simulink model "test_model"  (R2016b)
settings: Solver=VariableStepAuto  StartTime=0.0  StopTime=runtime  RelTol=1e-3
InitFcn:
  | clear mex
  | delete test_model_sfun.mexw64
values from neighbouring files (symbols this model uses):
  delta_T = 4 * [ 0,  0,  2.351e-4 ]    [modelParameters.m]
  Delta_T = cell(1,4)    [modelParameters.m]
  F_D = 1*randn(3,1)    [modelParameters.m]
  g = 9.81    [modelParameters.m]    (also in analyzeIMU_data.m = 9.8; getMomentOfInertia.m = 9.80665)
  Gamma_H = cell(1,4)    [modelParameters.m]
  have_motor_transient = 1    [modelParameters.m]
  height_controlled_o = (((Rm*If        + (((omega0_o * 2 * Rm * Kv * Kq      * Kd + 1)^2) - 1)/(4* Rm*Kv^2*Kq      * Kd))/Vb)*(Pmax - Pmin) + Pmin)    [modelParameters.m]
  i_0 = cell(1,4)    [modelParameters.m]
  If = 0.3836    [modelParameters.m]    (also in thrustDragConstantCalculations.m = [If0; If1; If2; If3]; Kd_error.m = I_0 * sign(rotor_speed_0) + I_1 * rotor_speed_0 + I_2 * roto)
  J = diag([ 0.0130 0.0140 0.0285 ])    [modelParameters.m]    (also in J_calc_bifilar.m = (16*pi^2*L./(m*g.*D.^2))\(t./n).^2)
  J_L = m_L/12*diag([y_L^2+z_L^2,x_L^2+z_L^2,x_L^2+y_L^2])    [modelParameters.m]
  J_r = cell(1,4)    [modelParameters.m]
  Jreq = 4.2012e-05    [modelParameters.m]
  Jxx = 0.0130    (= 0.013)    [modelParameters.m]
  Jyy = 0.0140    (= 0.014)    [modelParameters.m]
  Jzz = 0.0285    [modelParameters.m]
  K_d = cell(1,4)    [modelParameters.m]
  K_E = cell(1,4)    [modelParameters.m]
  K_H = cell(1,4)    [modelParameters.m]
  K_Q = cell(1,4)    [modelParameters.m]
  K_T = cell(1,4)    [modelParameters.m]
  K_V = cell(1,4)    [modelParameters.m]
  Kd = 1.4852e-07    [modelParameters.m]    (also in calcDragConstant.m = ((A'*A)^-1)*A'*b; thrustDragConstantCalculations.m = calcDragConstant(data, Pmin, Pmax, Rm, Kv, Kq, If); Kd_error.m = 1.0317e-07)
  Kh = 3.4574e-04    (= 0.00034574)    [modelParameters.m]
  Ki_mahony = 0.001    [modelParameters.m]
  Kp_mahony = 0.4    [modelParameters.m]
  Kq = 96.3422    [modelParameters.m]    (also in thrustDragConstantCalculations.m; Kd_error.m)
  Kt = 1.2007e-05    [modelParameters.m]    (also in calcThrustConstant.m = ((A'*A)^(-1))*(A'*T); thrustDragConstantCalculations.m = calcThrustConstant(data))
  Kv = 96.3422    [modelParameters.m]    (also in thrustDragConstantCalculations.m; Kd_error.m)
  m = 1.216    [modelParameters.m]
  m_L = 0    [modelParameters.m]
  omega0_o = sqrt((m*g)/(4*Kt))    [modelParameters.m]
  omega1_o = sqrt((m*g)/(4*Kt))    [modelParameters.m]
  omega2_o = sqrt((m*g)/(4*Kt))    [modelParameters.m]
  omega3_o = sqrt((m*g)/(4*Kt))    [modelParameters.m]
  omega_0 = cell(1,4)    [modelParameters.m]
  p0 = 0    [modelParameters.m]
  p_0 = cell(1,4)    [modelParameters.m]
  p_max = cell(1,4)    [modelParameters.m]
  phi0 = 0    [modelParameters.m]
  pitch_o = 0    [modelParameters.m]
  pitchrate_o = 0    [modelParameters.m]
  Pmax = 1    [modelParameters.m]    (also in thrustDragConstantCalculations.m = 200000; Kd_error.m = 200000)
  Pmin = 0    [modelParameters.m]    (also in thrustDragConstantCalculations.m = 100000; Kd_error.m = 100000)
  psi0 = 0    [modelParameters.m]
  q0 = 0    [modelParameters.m]
  Q_D = 0.05*randn(3,1)    [modelParameters.m]
  r0 = 0    [modelParameters.m]
  R_m = cell(1,4)    [modelParameters.m]
  r_oc = [ 0 ; 0 ; 0 ]    [modelParameters.m]
  r_oL = [0; 0; 0]    [modelParameters.m]
  rhx = 0.16    [modelParameters.m]
  rhy = 0.16    [modelParameters.m]
  rhz = 0.03    [modelParameters.m]
  Rm = 0.235    [modelParameters.m]    (also in thrustDragConstantCalculations.m = 0.2308; Kd_error.m = 0.2308)
  roll_o = 0    [modelParameters.m]
  rollrate_o = 0    [modelParameters.m]
  Tc = 0.04    [modelParameters.m]
  theta0 = 0    [modelParameters.m]
  Tq = 0.005    [modelParameters.m]
  u0 = 0    [modelParameters.m]
  v0 = 0    [modelParameters.m]
  Vb = 12.3    [modelParameters.m]    (also in calcDragConstant.m = [data.(6); data.(6); data.(6); data.(6)]; Kd_error.m = data.(6))
  w0 = 0    [modelParameters.m]
  x0 = 0    [modelParameters.m]
  x_controlled_o = 0    [modelParameters.m]
  x_o = 0    [modelParameters.m]
  x_vel_o = 0    [modelParameters.m]
  y0 = 0    [modelParameters.m]
  y_controlled_o = 0    [modelParameters.m]
  y_o = 0    [modelParameters.m]
  y_vel_o = 0    [modelParameters.m]
  yaw_controlled_o = 0    [modelParameters.m]
  yaw_o = 0    [modelParameters.m]
  yawrate_o = 0    [modelParameters.m]
  z0 = 0    [modelParameters.m]
  z_o = 0    [modelParameters.m]
  z_vel_o = 0    [modelParameters.m]
undefined symbols (not defined in the file or in its folder): Gamma_Omega, Gamma_T, Ki, Kp, r_h, slope, start, Ts, X0
libraries: simulink x32, Derivative x26, dsparch4 x6, vrlib x4
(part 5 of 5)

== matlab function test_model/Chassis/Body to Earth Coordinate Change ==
function x_E = body2earth(x_B,Theta)
%#codegen

phi = Theta(1); 
theta = Theta(2); 
psi = Theta(3); 

L_BE = [ cos(theta)*cos(psi) , sin(phi)*sin(theta)*cos(psi)-cos(phi)*sin(psi) , cos(phi)*sin(theta)*cos(psi)+sin(phi)*sin(psi) ; 
         cos(theta)*sin(psi) , sin(phi)*sin(theta)*sin(psi)+cos(phi)*cos(psi) , cos(phi)*sin(theta)*sin(psi)-sin(phi)*cos(psi) ; 
                 -sin(theta) ,                            sin(phi)*cos(theta) , cos(phi)*cos(theta) ];
x_E = L_BE*x_B; 

end

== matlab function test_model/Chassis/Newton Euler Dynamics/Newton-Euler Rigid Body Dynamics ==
function [dv,dOmega] = newton_euler(F,Q,v,Omega,m,J,r_oc)
%#codegen 

r_oc_X = [ 0 -r_oc(3) r_oc(2) ; r_oc(3) 0 -r_oc(1) ; -r_oc(2) r_oc(1) 0 ]; 

M = [ m*eye(3) , -m*r_oc_X ; 
    zeros(3,3) , J ];

f = M^-1*[F - m*cross(Omega,v) - m*cross(Omega,cross(Omega,r_oc)) ; ... 
          Q - cross(Omega,J*Omega) - cross(r_oc,F) ];

dv = f(1:3); 
dOmega = f(4:6); 

end

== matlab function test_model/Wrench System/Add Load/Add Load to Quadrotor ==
function [m,J,r_oc] = add_load(m_0,J_0,r_oc_0,m_l,J_l,r_ol)
%#codegen
r_oc = (m_0*r_oc_0 + m_l*r_ol)/(m_0+m_l); 
m = m_0 + m_l; 
r_cl = -r_oc + r_ol; 
r_co = -r_oc; 
J = J_0 + J_l + m_0*(r_co'*r_co*eye(3) - r_co*r_co') + m_l*(r_cl'*r_cl*eye(3) - r_cl*r_cl'); 

end

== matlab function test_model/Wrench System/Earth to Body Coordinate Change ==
function x_B = earth2body(x_E,Theta)
%#codegen

phi = Theta(1); 
theta = Theta(2); 
psi = Theta(3); 

             
L_EB = [                           cos(theta)*cos(psi) ,                            cos(theta)*sin(psi) ,         -sin(theta) ; 
        sin(phi)*sin(theta)*cos(psi)-cos(phi)*sin(psi) , sin(phi)*sin(theta)*sin(psi)+cos(phi)*cos(psi) , sin(phi)*cos(theta) ; 
        cos(phi)*sin(theta)*cos(psi)+sin(phi)*sin(psi) , cos(phi)*sin(theta)*sin(psi)-sin(phi)*cos(psi) , cos(phi)*cos(theta)]; 

x_B = L_EB*x_E;  

end

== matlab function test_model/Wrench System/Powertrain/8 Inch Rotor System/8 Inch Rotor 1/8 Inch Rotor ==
function [F,Q] = rotor_8_inch(omega,alpha,v,Omega,K_T,K_H,K_d,r_h,Delta_T,Gamma_T,Gamma_H,Gamma_Omega,J_r)
%#codegen

% calculate hub velocity
v_h = v + cross(Omega,r_h); 

% calculate thrust
%T = K_T*(omega^2)*Gamma_T;
T = (K_T*(omega^2) + Delta_T'*v_h*omega)*Gamma_T;
% calculate H force
H = -K_H*omega*Gamma_H*v_h; %[-v(1);-v(2);-0.5*v(3)];

% calculate total force
F = T + H; 

% calculate force lever-arm torque 
Q_F = cross(r_h,F); 
% calculate drag torque 
Q_d = -K_d*(omega^2)*Gamma_Omega; 
% calculate gyroscopic torque 
Q_g = -cross( J_r*Omega, omega*Gamma_Omega ); 
% calculate in plane acceleration torque
Q_a = -J_r*alpha*Gamma_Omega; 
% produce torque vector
Q = Q_F + Q_d + Q_g + Q_a; 

end

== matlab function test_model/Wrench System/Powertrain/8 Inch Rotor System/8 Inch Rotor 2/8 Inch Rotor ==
function [F,Q] = rotor_8_inch(omega,alpha,v,Omega,K_T,K_H,K_d,r_h,Delta_T,Gamma_T,Gamma_H,Gamma_Omega,J_r)
%#codegen

% calculate hub velocity
v_h = v + cross(Omega,r_h); 

% calculate thrust
% T = K_T*(omega^2)*Gamma_T;
T = (K_T*(omega^2) + Delta_T'*v_h*omega)*Gamma_T;

% calculate H force
H = -K_H*omega*Gamma_H*v_h; %[-v(1);-v(2);-0.5*v(3)];

% calculate total force
F = T + H; 

% calculate force lever-arm torque 
Q_F = cross(r_h,F); 
% calculate drag torque 
Q_d = -K_d*(omega^2)*Gamma_Omega; 
% calculate gyroscopic torque 
Q_g = -cross( J_r*Omega, omega*Gamma_Omega ); 
% calculate in plane acceleration torque
Q_a = -J_r*alpha*Gamma_Omega; 
% produce torque vector
Q = Q_F + Q_d + Q_g + Q_a; 

end

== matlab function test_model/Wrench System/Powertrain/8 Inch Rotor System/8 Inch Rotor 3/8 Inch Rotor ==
function [F,Q] = rotor_8_inch(omega,alpha,v,Omega,K_T,K_H,K_d,r_h,Delta_T,Gamma_T,Gamma_H,Gamma_Omega,J_r)
%#codegen

% calculate hub velocity
v_h = v + cross(Omega,r_h); 

% calculate thrust
%T = K_T*(omega^2)*Gamma_T;
T = (K_T*(omega^2) + Delta_T'*v_h*omega)*Gamma_T;
% calculate H force
H = -K_H*omega*Gamma_H*v_h; %[-v(1);-v(2);-0.5*v(3)];

% calculate total force
F = T + H; 

% calculate force lever-arm torque 
Q_F = cross(r_h,F); 
% calculate drag torque 
Q_d = -K_d*(omega^2)*Gamma_Omega; 
% calculate gyroscopic torque 
Q_g = -cross( J_r*Omega, omega*Gamma_Omega ); 
% calculate in plane acceleration torque
Q_a = -J_r*alpha*Gamma_Omega; 
% produce torque vector
Q = Q_F + Q_d + Q_g + Q_a; 

end

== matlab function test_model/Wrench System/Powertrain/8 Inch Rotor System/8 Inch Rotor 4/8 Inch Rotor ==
function [F,Q] = rotor_8_inch(omega,alpha,v,Omega,K_T,K_H,K_d,r_h,Delta_T,Gamma_T,Gamma_H,Gamma_Omega,J_r)
%#codegen

% calculate hub velocity
v_h = v + cross(Omega,r_h); 

% calculate thrust
%T = K_T*(omega^2)*Gamma_T;
T = (K_T*(omega^2) + Delta_T'*v_h*omega)*Gamma_T;
% calculate H force
H = -K_H*omega*Gamma_H*v_h; %[-v(1);-v(2);-0.5*v(3)];

% calculate total force
F = T + H; 

% calculate force lever-arm torque 
Q_F = cross(r_h,F); 
% calculate drag torque 
Q_d = -K_d*(omega^2)*Gamma_Omega; 
% calculate gyroscopic torque 
Q_g = -cross( J_r*Omega, omega*Gamma_Omega ); 
% calculate in plane acceleration torque
Q_a = -J_r*alpha*Gamma_Omega; 
% produce torque vector
Q = Q_F + Q_d + Q_g + Q_a; 

end

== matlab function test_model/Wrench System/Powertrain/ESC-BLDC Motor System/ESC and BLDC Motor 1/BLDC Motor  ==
function alpha = BLDC_motor(V,omega,R_m,K_Q,K_V,i_0,K_d,J_r)
%#codegen
alpha = 1/J_r*(V/(R_m*K_Q)-omega/(R_m*K_Q*K_V)-sign(omega)*i_0/K_Q-K_d*omega^2);
end

== matlab function test_model/Wrench System/Powertrain/ESC-BLDC Motor System/ESC and BLDC Motor 1/BLDC Motor 
(no transient) ==
function [alpha,omega] = BLDC_motor_no_transient(V,R_m,K_Q,K_V,i_0,K_d)
%#codegen
alpha = 0;
omega = (-1 + sqrt(1-4*R_m*K_d*K_Q*K_V*(K_V*R_m*i_0-K_V*V)))/(2*R_m*K_d*K_Q*K_V); 
% omega = 50.7815*(V-6.749)+470.0908; 
end

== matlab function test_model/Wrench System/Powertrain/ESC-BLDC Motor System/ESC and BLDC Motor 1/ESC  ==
function V = esc_cmd(p,V_b,K_E,p_0,p_max)
%#codegen

u_p = (p - p_0)/(p_max - p_0);

V = K_E*u_p*V_b; 

end

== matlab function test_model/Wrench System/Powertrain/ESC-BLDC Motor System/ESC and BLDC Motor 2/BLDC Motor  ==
function alpha = BLDC_motor(V,omega,R_m,K_Q,K_V,i_0,K_d,J_r)
%#codegen
alpha = 1/J_r*(V/(R_m*K_Q)-omega/(R_m*K_Q*K_V)-sign(omega)*i_0/K_Q-K_d*omega^2);
end

== matlab function test_model/Wrench System/Powertrain/ESC-BLDC Motor System/ESC and BLDC Motor 2/BLDC Motor 
(no transient) ==
function [alpha,omega] = BLDC_motor_no_transient(V,R_m,K_Q,K_V,i_0,K_d)
%#codegen
alpha = 0;
omega = (-1 + sqrt(1-4*R_m*K_d*K_Q*K_V*(K_V*R_m*i_0-K_V*V)))/(2*R_m*K_d*K_Q*K_V); 
% omega = 50.7815*(V-6.749)+470.0908; 
end

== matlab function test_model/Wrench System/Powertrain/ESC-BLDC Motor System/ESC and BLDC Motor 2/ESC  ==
function V = esc_cmd(p,V_b,K_E,p_0,p_max)
%#codegen

u_p = (p - p_0)/(p_max - p_0);

V = K_E*u_p*V_b; 

end

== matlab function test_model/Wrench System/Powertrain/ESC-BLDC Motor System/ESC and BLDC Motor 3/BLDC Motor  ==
function alpha = BLDC_motor(V,omega,R_m,K_Q,K_V,i_0,K_d,J_r)
%#codegen
alpha = 1/J_r*(V/(R_m*K_Q)-omega/(R_m*K_Q*K_V)-sign(omega)*i_0/K_Q-K_d*omega^2);
end

== matlab function test_model/Wrench System/Powertrain/ESC-BLDC Motor System/ESC and BLDC Motor 3/BLDC Motor 
(no transient) ==
function [alpha,omega] = BLDC_motor_no_transient(V,R_m,K_Q,K_V,i_0,K_d)
%#codegen
alpha = 0;
omega = (-1 + sqrt(1-4*R_m*K_d*K_Q*K_V*(K_V*R_m*i_0-K_V*V)))/(2*R_m*K_d*K_Q*K_V); 
% omega = 50.7815*(V-6.749)+470.0908; 
end

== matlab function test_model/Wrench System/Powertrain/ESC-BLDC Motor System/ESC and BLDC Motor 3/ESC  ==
function V = esc_cmd(p,V_b,K_E,p_0,p_max)
%#codegen

u_p = (p - p_0)/(p_max - p_0);

V = K_E*u_p*V_b; 

end

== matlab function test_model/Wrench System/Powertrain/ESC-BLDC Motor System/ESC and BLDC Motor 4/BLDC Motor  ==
function alpha = BLDC_motor(V,omega,R_m,K_Q,K_V,i_0,K_d,J_r)
%#codegen
alpha = 1/J_r*(V/(R_m*K_Q)-omega/(R_m*K_Q*K_V)-sign(omega)*i_0/K_Q-K_d*omega^2);
end

== matlab function test_model/Wrench System/Powertrain/ESC-BLDC Motor System/ESC and BLDC Motor 4/BLDC Motor 
(no transient) ==
function [alpha,omega] = BLDC_motor_no_transient(V,R_m,K_Q,K_V,i_0,K_d)
%#codegen
alpha = 0;
omega = (-1 + sqrt(1-4*R_m*K_d*K_Q*K_V*(K_V*R_m*i_0-K_V*V)))/(2*R_m*K_d*K_Q*K_V); 
% omega = 50.7815*(V-6.749)+470.0908; 
end

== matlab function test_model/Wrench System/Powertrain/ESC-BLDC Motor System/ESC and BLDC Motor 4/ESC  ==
function V = esc_cmd(p,V_b,K_E,p_0,p_max)
%#codegen

u_p = (p - p_0)/(p_max - p_0);

V = K_E*u_p*V_b; 

end

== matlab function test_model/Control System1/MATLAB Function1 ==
function [z_corr, y_cor, x_corr, yaw_corr, pid_y_out, pid_roll_out] = c_controller(set_x, set_y, set_z, set_yaw, ...
    cur_x, cur_y, cur_z, ...
    cur_phi, cur_theta, cur_psi, ...
    cur_phi_d, cur_theta_d, cur_psi_d, vrpn_id, Tc)

out_z = -1;
out_y = -1;
out_x = -1;
out_yaw = -1;
c_pid_y = -1;
c_pid_roll = -1;

coder.ceval('c_controller', vrpn_id, Tc, set_x, set_y, set_z, set_yaw, ...
                    cur_x, cur_y, cur_z, ...
                    cur_phi, cur_theta, cur_psi, ...
                    cur_phi_d, cur_theta_d, cur_psi_d, ...
                    coder.wref(out_z), coder.wref(out_y), coder.wref(out_x), coder.wref(out_yaw), ...
                    coder.wref(c_pid_y), coder.wref(c_pid_roll));

z_corr = out_z;
y_cor = out_y;
x_corr = out_x;
pid_y_out = c_pid_y;
pid_roll_out = c_pid_roll;
yaw_corr = out_yaw;

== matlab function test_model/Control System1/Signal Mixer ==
function P  = signal_mixer(height_controlled, y_controlled, x_controlled, yaw_controlled)

controller_outputs = [ height_controlled; x_controlled; y_controlled; yaw_controlled ];
signal_mixer = [ 1, -1, -1, -1; ... 
                 1,  1, -1,  1; ...
                 1, -1,  1,  1; ...
                 1,  1,  1, -1 ];
             
P = signal_mixer * controller_outputs;

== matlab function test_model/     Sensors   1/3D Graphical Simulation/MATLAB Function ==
function y = eigenaxis_ucart(u)


if abs(u(1))< 0.0001
    u(1) = 0.0001;
end

if abs(u(2))< 0.0001
    u(2) = 0.0001;
end

if abs(u(3))< 0.0001
    u(3) = 0.0001;
end

u = [ -u(1); -u(2); u(3) ];% [Pitch, Yaw, Roll] 

C11 = cos(u(2))*cos(u(3));
C12 = cos(u(2))*sin(u(3));
C13 = -sin(u(2));
C21 = sin(u(1))*sin(u(2))*cos(u(3))-cos(u(1))*sin(u(3));
C22 = sin(u(1))*sin(u(2))*sin(u(3))+cos(u(1))*cos(u(3));
C23 = sin(u(1))*cos(u(2));
C31 = cos(u(1))*sin(u(2))*cos(u(3))+sin(u(1))*sin(u(3));
C32 = cos(u(1))*sin(u(2))*sin(u(3))-sin(u(1))*cos(u(3));
C33 = cos(u(1))*cos(u(2));
    
theta = acos(0.5*(C11+C22+C33-1));

e = [C23-C32; C31-C13; C12-C21]/(2*sin(theta));
    
y = [e; theta];

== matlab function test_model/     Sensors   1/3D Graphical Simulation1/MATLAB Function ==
function y = eigenaxis_ucart(u)


if abs(u(1))< 0.0001
    u(1) = 0.0001;
end

if abs(u(2))< 0.0001
    u(2) = 0.0001;
end

if abs(u(3))< 0.0001
    u(3) = 0.0001;
end

u = [ -u(1); -u(2); u(3) ];% [Pitch, Yaw, Roll] 

C11 = cos(u(2))*cos(u(3));
C12 = cos(u(2))*sin(u(3));
C13 = -sin(u(2));
C21 = sin(u(1))*sin(u(2))*cos(u(3))-cos(u(1))*sin(u(3));
C22 = sin(u(1))*sin(u(2))*sin(u(3))+cos(u(1))*cos(u(3));
C23 = sin(u(1))*cos(u(2));
C31 = cos(u(1))*sin(u(2))*cos(u(3))+sin(u(1))*sin(u(3));
C32 = cos(u(1))*sin(u(2))*sin(u(3))-sin(u(1))*cos(u(3));
C33 = cos(u(1))*cos(u(2));
    
theta = acos(0.5*(C11+C22+C33-1));

e = [C23-C32; C31-C13; C12-C21]/(2*sin(theta));
    
y = [e; theta];

== matlab function test_model/     Sensors   1/Aeb









 ==
function euler_rates_IMU = angular_body_earth_conversion(gyro_reading, euler_angles_filtered)

phi = euler_angles_filtered(1);
theta = euler_angles_filtered(2);

Aeb = [1, sin(phi)*tan(theta), cos(phi)*tan(theta); ...
       0,     cos(phi)       ,        -sin(phi)   ; ...
       0,  sin(phi)/cos(theta), cos(phi)/cos(theta)];

   
euler_rates_IMU = Aeb * gyro_reading;

== matlab function test_model/     Sensors   1/Aeb_c









1 ==
function euler_rates_IMU = angular_body_earth_conversion(gyro_reading, euler_angles_filtered)

phi = euler_angles_filtered(1);
theta = euler_angles_filtered(2);
psi = NaN;

phi_dot = -1;
theta_dot = -1;
psi_dot = -1;

p = gyro_reading(1);
q = gyro_reading(2);
r = gyro_reading(3);

coder.ceval( 'aeb_mat', p, q, r, phi, theta, psi, coder.wref(phi_dot), ...
    coder.wref(theta_dot), coder.wref(psi_dot) );

   
euler_rates_IMU = [phi_dot; theta_dot; psi_dot];

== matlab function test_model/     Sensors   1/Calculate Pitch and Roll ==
function [accel_pitch, accel_roll] = getPitchAndRoll(accel_reading)

x_accel = accel_reading(1);
y_accel = accel_reading(2);
z_accel = accel_reading(3);

accel_pitch = atan(x_accel/sqrt(y_accel^2 + z_accel^2));
accel_roll = atan( -y_accel/( sqrt(z_accel^2 + x_accel^2))  );

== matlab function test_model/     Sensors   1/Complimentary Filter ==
function euler_angles_IMU   = complimentaryFilter(accel_pitch, accel_roll, euler_rates_gyro, prev_euler_angles)

k_gyro = 0.99; 
k_accel = 1-k_gyro; 

Ts = 0.005; % 5 milliseconds

prev_phi = prev_euler_angles(1);
prev_theta = prev_euler_angles(2);

prev_phi_dot = euler_rates_gyro(1);
prev_theta_dot = euler_rates_gyro(2);

integrated_phi_gyro = Ts * prev_phi_dot + prev_phi;
integrated_theta_gyro = Ts * prev_theta_dot + prev_theta;

phi = k_gyro * integrated_phi_gyro + k_accel * accel_roll;
theta = k_gyro * integrated_theta_gyro + k_accel * accel_pitch;

euler_angles_IMU = [phi; theta];

== matlab function test_model/     Sensors   1/IMU





/






 ==
function [accelReading,gyroReading] = idealIMU(B_vo_dot, B_vo, B_Omega, B_g, g, r_oc)
%#codegen

a = B_vo_dot + cross(B_Omega,B_vo); % body frame acceleration 

accelReading = (a - B_g)/g ; % accelerometer reading (ideal)

gyroReading = B_Omega ; % gyroscope reading (ideal) 

end

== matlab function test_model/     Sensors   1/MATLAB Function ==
function euler_angles_IMU  = complimentaryFilterC(accel_pitch, accel_roll, euler_rates_gyro)

euler_x = euler_rates_gyro(1);
euler_y = euler_rates_gyro(2);

filtered_pitch = -1;
filtered_roll = -1;

coder.ceval('compl_filter', accel_pitch, accel_roll, euler_x, euler_y, ...
            coder.wref(filtered_pitch), coder.wref(filtered_roll));

euler_angles_IMU = [filtered_roll; filtered_pitch];

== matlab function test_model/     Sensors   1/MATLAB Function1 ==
function [accel_pitch, accel_roll]  = angle_IMU_C(accel_reading)

accel_x = accel_reading(1);
accel_y = accel_reading(2);
accel_z = accel_reading(3);

calculated_pitch = -1;
calculated_roll = -1;

coder.ceval('angle_accel', accel_x, accel_y, accel_z, coder.wref(calculated_pitch), coder.wref(calculated_roll));

accel_pitch = calculated_pitch;
accel_roll = calculated_roll;

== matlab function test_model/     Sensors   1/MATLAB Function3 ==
function [eulerAngles, integralFeedback, quaternions] = ...
    mahonyFilter(accelReadings, gyroReadings, quaternions_prev, ...
    integralFeedback_prev, Tq, Kp_mahony, Ki_mahony)
%     mahonyFilter(accelReadings, gyroReadings, eulerAngles_prev, ...
%     integralFeedback_prev, Tq, Kp_mahony, Ki_mahony)
    
    
    %Save quadcopter loop time as dt
    dt = Tq;

    %Pull accelerometer readings and negate them to compare
    accel_x = accelReadings(1);
    accel_y = accelReadings(2);
    accel_z = accelReadings(3);
    
    %Negate the accelerometer values to compare with direction of the
    %gravity vector
    accel_x = (-1) * accel_x;
    accel_y = (-1) * accel_y;
    accel_z = (-1) * accel_z;

    %Pull gyroscope readings
    gyro_x = gyroReadings(1);
    gyro_y = gyroReadings(2);
    gyro_z = gyroReadings(3);

    %Pull previous Euler angles
%     roll_prev = eulerAngles_prev(1);
%     pitch_prev = eulerAngles_prev(2);
%     yaw_prev = eulerAngles_prev(3);
    
    %Pull previous integral feedback terms
    integralFeedback_x_prev = integralFeedback_prev(1);
    integralFeedback_y_prev = integralFeedback_prev(2);
    integralFeedback_z_prev = integralFeedback_prev(3);

    %Calculate half cosines and sines for the quaternion elements
%     cosHalfRoll = cos( 0.5 * roll_prev );
%     sinHalfRoll = sin( 0.5 * roll_prev );
%     cosHalfPitch = cos( 0.5 * pitch_prev );
%     sinHalfPitch = sin( 0.5 * pitch_prev );
%     cosHalfYaw = cos( 0.5 * yaw_prev );
%     sinHalfYaw = sin( 0.5 * yaw_prev );

    %Calculate the quaternion elements
%     q0 = cosHalfRoll * cosHalfPitch * cosHalfYaw + ...
%         sinHalfRoll * sinHalfPitch * sinHalfYaw;
% 
%     q1 = sinHalfRoll * cosHalfPitch * cosHalfYaw - ...
%         cosHalfRoll * sinHalfPitch * sinHalfYaw;
% 
%     q2 = cosHalfRoll * sinHalfPitch * cosHalfYaw + ...
%         sinHalfRoll * cosHalfPitch * sinHalfYaw;
% 
%     q3 = (-1) * sinHalfRoll * sinHalfPitch * cosHalfYaw + ...
%         cosHalfRoll * cosHalfPitch * sinHalfYaw;

    %Pull the quaternion values
    q0 = quaternions_prev(1);
    q1 = quaternions_prev(2);
    q2 = quaternions_prev(3);
    q3 = quaternions_prev(4);


    %Calculate the rate of change of the quaternion from the gyroscope
%     q0_dot = 0.5 * ( (-1)*(q1 * gyro_x) - (q2 * gyro_y) - (q3 * gyro_z) );
%     q1_dot = 0.5 * ( (q0 * gyro_x) + (q2 * gryo_z) - (q3 * gyro_y) );
%     q2_dot = 0.5 * ( (q0 * gyro_y) - (q1 * gyro_z) + (q3 * gyro_x) );
%     q3_dot = 0.5 * ( (q0 * gyro_z) + (q1 * gyro_y) - (q2 * gyro_x) );

    %Define initial values for the corrected gyroscope values
    gyro_x_corrected = gyro_x;
    gyro_y_corrected = gyro_y;
    gyro_z_corrected = gyro_z;
    
    %Define initial values for the corrected integral feedback values
    integralFeedback_x = integralFeedback_x_prev;
    integralFeedback_y = integralFeedback_y_prev;
    integralFeedback_z = integralFeedback_z_prev;

    %Only compute the feedback if the accelerometer measurements are valid
    %This prevents NaN values when normalizing the accelerometer measurements
    if( accel_x ~= 0 && accel_y ~= 0  && accel_z ~= 0 )

       %Check... maybe we don't need to do this normalization...
       %Ideally our accelerometer readings should have a magnitude of 1, but
       %this is usually not the case with data we have collected
       accel_mag = ( (accel_x ^ 2) + (accel_y ^ 2) + (accel_z ^ 2) ) ^ 0.5;
       accel_x = accel_x / accel_mag;
       accel_y = accel_y / accel_mag;
       accel_z = accel_z / accel_mag;

       %Estimate direction of gravity
       vx = 2 * ( (q1 * q3) - (q0 * q2) );
       vy = 2 * ( (q0 * q1) + (q2 * q3) );
       vz = (2 * q0 * q0) - (q3 * q3);
       
       %Error is the sum of the cross product between the estimated and
       %measured direction of gravity
       ex = (accel_y * vz) - (accel_z * vy);
       ey = (accel_z * vx) - (accel_x * vz);
       ez = (accel_x * vy) - (accel_y * vx);
       
       %Compute and apply the proportional feedback
       gyro_x_corrected = gyro_x + (Kp_mahony * ex);
       gyro_y_corrected = gyro_y + (Kp_mahony * ey);
       gyro_z_corrected = gyro_z + (Kp_mahony * ez);

       %Compute and apply the integral feedback, if it is enabled
       if ( Ki_mahony > 0 )
           
           %Integrate digitally based on sample time and scale by Ki, and
           %accumulate the integral term by adding this to the previous
           %feedback term
           integralFeedback_x = (Ki_mahony * ex * dt) + ...
               integralFeedback_x_prev;
           integralFeedback_y = (Ki_mahony * ey * dt) + ...
               integralFeedback_y_prev;
           integralFeedback_z = (Ki_mahony * ez * dt) + ...
               integralFeedback_z_prev;
           
           %Correct the gyroscope values using the new integral feedback
           gyro_x_corrected = gyro_x_corrected + integralFeedback_x;
           gyro_y_corrected = gyro_y_corrected + integralFeedback_y;
           gyro_z_corrected = gyro_z_corrected + integralFeedback_z;
           
       else
           
           %Otherwise, reset the integral terms to zero to prevent windup
           integralFeedback_x = 0;
           integralFeedback_y = 0;
           integralFeedback_z = 0;
           
       end %if ( Ki_mahoney > 0 )

    end %if ( accel_x ~= 0 && accel_y ~= 0 && accel_z ~= 0 )

    %Integrate the rate of change of the quaternion
    %First, pre-multiply the common factors to the gyro reading values
    gyro_x_corrected = gyro_x_corrected * (0.5 * dt);
    gyro_y_corrected = gyro_y_corrected * (0.5 * dt);
    gyro_z_corrected = gyro_z_corrected * (0.5 * dt);
    
    %Now, create temporary variales for the first three quaternion values
    qa = q0;
    qb = q1;
    qc = q2;
    
    %Now perform calculation to integrate the rate of the quaternion
    q0 = q0 - (qb * gyro_x_corrected) - (qc * gyro_y_corrected) - ...
        (q3 * gyro_z_corrected);
    q1 = q1 + (qa * gyro_x_corrected) + (qc * gyro_z_corrected) - ...
        (q3 * gyro_y_corrected);
    q2 = q2 + (qa * gyro_y_corrected) - (qb * gyro_z_corrected) + ...
        (q3 * gyro_x_corrected);
    q3 = q3 + (qa * gyro_z_corrected) + (qb * gyro_y_corrected) - ...
        (qc * gyro_x_corrected);
    
    %Normalize quaternion
    quaternion_mag = ( (q0 * q0) + (q1 * q1) + (q2 * q2) + (q3 * q3) ) ^ 0.5;
    q0 = q0 / quaternion_mag;
    q1 = q1 / quaternion_mag;
    q2 = q2 / quaternion_mag;
    q3 = q3 / quaternion_mag;
    
    %Estimate the gravity direction from the quaternion values
    grav_x = 2 * ( (q1 * q3) - (q0 * q2) );
    grav_y = 2 * ( (q0 * q1) + (q2 * q3) );
    grav_z = (q0 * q0) - (q1 * q1) - (q2 * q2) + (q3 * q3);
    
    %Limit the gravity vector in x-direction to maintain a magnitude of 1
%     grav_x = min( grav_x , 1 );
%     grav_x = max( grav_x , -1 );

    %Normalize the gravity vector
    grav_mag = sqrt( ( grav_x * grav_x ) + ( grav_y * grav_y ) + ...
        ( grav_z * grav_z ) );
    grav_x = grav_x / grav_mag;
    grav_y = grav_y / grav_mag;
    grav_z = grav_z / grav_mag;
    
    %Calculate the pitch, roll, and yaw
    yaw = atan2( 2 * ( (q0 * q3) + (q1 * q2) ) , ...
        (q0 * q0) + (q1 * q1) - (q2 * q2) - (q3 * q3) );
    pitch = asin( (-1) * grav_x );
    roll = atan2( grav_y , grav_z );
    
    %Create a vector of current integral feedback terms to output
    integralFeedback = [ integralFeedback_x ; ...
        integralFeedback_y ; integralFeedback_z ];
    
    %Create a vector of the corrected gyroscope terms
    %gyroReadings_corrected = [ gyro_x_corrected ; ...
    %    gyro_y_corrected ; gyro_z_corrected ];
    
    %Create a vector of the newly calculated quaternion values
    quaternions = [ q0 ; q1 ; q2 ; q3 ];
    
    %Create a vector of the calculated Euler angles
    eulerAngles = [ roll ;  pitch ; yaw ];
    
end %function

== matlab function test_model/Control System/Controller/Pseudo-Nonlinear Extension









1 ==
function [phi_setpoint_corrected, theta_setpoint_corrected] = pseudo_nonlinear_extension(phi_setpoint, theta_setpoint, yaw)
phi_setpoint_corrected = theta_setpoint * cos(yaw) - phi_setpoint * sin(yaw);
theta_setpoint_corrected = theta_setpoint * sin(yaw) + phi_setpoint * cos(yaw);
end
